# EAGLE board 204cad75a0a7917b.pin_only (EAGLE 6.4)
REV: B

Size 50.8 x 22.86 mm. Coordinates in mm from the lower left corner, seen from the top.
Outline: 2.54,0 48.26,0 arc90 50.8,2.54 50.8,20.32 arc90 48.26,22.86 2.54,22.86 arc90 0,20.32 0,13.97 0.51,13.46 0.51,9.4 0,8.89 0,2.54 arc90 2.54,0
Copper layers (1*16): Top 0.035mm / dielectric 1.5mm / Bottom 0.035mm
Design rules "adafruit *": minimum track width 8mil, minimum drill 15.5mil, track to track 8mil, track to pad 8mil, pad to pad 8mil, via to via 8mil, smd to smd 8mil, copper to edge 10mil, drill to drill 8mil, minimum pad ring 10mil, minimum via ring 8mil, stop-mask expansion 2mil, vias tented up to drill 20mil, thermal gap 10mil
Holes 2.54 mm at 48.26,20.32 48.26,2.54
tRestrict: area 20.8,9.3 to 21.1,12.8; area 20.7,8.1 to 22.9,8.5; area 26.2,10.3 to 26.5,13.3

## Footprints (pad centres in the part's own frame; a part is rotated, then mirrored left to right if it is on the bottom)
1X01_ROUND = drill 1 pad 1.676: 1 0,0
0805-NO = smd 1.24 x 1.5: 1 -0.95,0; 2 0.95,0
0603-NO = smd 1.1 x 1: 1 -0.85,0; 2 0.85,0
_0603MP = smd 0.8 x 0.8: 1 -0.762,0; 2 0.762,0
CHIPLED_0805_NOOUTLINE = smd 1.2 x 1.2: A 0,-1.05; C 0,1.05
SOD-123 = smd 1.4 x 1.4: A 1.85,0; C -1.85,0
TQFN44_7MM = smd 0.25 x 0.8: 1 -2.5,-3.475; 2 -2,-3.475; 3 -1.5,-3.475; 4 -1,-3.475; 5 -0.5,-3.475; 6 0,-3.475; 7 0.5,-3.475; 8 1,-3.475; 9 1.5,-3.475; 10 2,-3.475; 11 2.5,-3.475; 23 2.5,3.475; 24 2,3.475; 25 1.5,3.475; 26 1,3.475; 27 0.5,3.475; 28 0,3.475; 29 -0.5,3.475; 30 -1,3.475; 31 -1.5,3.475; 32 -2,3.475; 33 -2.5,3.475 | smd 0.8 x 0.25: 12 3.475,-2.5; 13 3.475,-2; 14 3.475,-1.5; 15 3.475,-1; 16 3.475,-0.5; 17 3.475,0; 18 3.475,0.5; 19 3.475,1; 20 3.475,1.5; 21 3.475,2; 22 3.475,2.5; 34 -3.475,2.5; 35 -3.475,2; 36 -3.475,1.5; 37 -3.475,1; 38 -3.475,0.5; 39 -3.475,0; 40 -3.475,-0.5; 41 -3.475,-1; 42 -3.475,-1.5; 43 -3.475,-2; 44 -3.475,-2.5 | smd 4.7 x 4.7: THERMAL 0,0
1X16_ROUND = drill 1 pad 1.676: 1 -19.05,0; 2 -16.51,0; 3 -13.97,0; 4 -11.43,0; 5 -8.89,0; 6 -6.35,0; 7 -3.81,0; 8 -1.27,0; 9 1.27,0; 10 3.81,0; 11 6.35,0; 12 8.89,0; 13 11.43,0; 14 13.97,0; 15 16.51,0; 16 19.05,0
1X12_ROUND = drill 1 pad 1.676: 1 -13.97,0; 2 -11.43,0; 3 -8.89,0; 4 -6.35,0; 5 -3.81,0; 6 -1.27,0; 7 1.27,0; 8 3.81,0; 9 6.35,0; 10 8.89,0; 11 11.43,0; 12 13.97,0
1X02_ROUND = drill 1 pad 1.778: 1 -1.27,0; 2 1.27,0
KMR2 = smd 1 x 1: 1 2,0.8; 2 2,-0.8; 3 -2,0.8; 4 -2,-0.8
SOT23-5 = smd 0.55 x 1.2: 1 -0.95,-1.3; 2 0,-1.3; 3 0.95,-1.3; 4 0.95,1.3; 5 -0.95,1.3
RFMHCW_SMT = smd 1.5 x 1: 1P 8.1,-7; 2P 8.1,-5; 3P 8.1,-3; 4P 8.1,-1; 5P 8.1,1; 6P 8.1,3; 7P 8.1,5; 8P 8.1,7; 9P -8.1,7; 10P -8.1,5; 11P -8.1,3; 12P -8.1,1; 13P -8.1,-1; 14P -8.1,-3; 15P -8.1,-5; 16P -8.1,-7
MOUNTINGHOLE_2.5_PLATED = drill 2.5 pad 3.2: P$1 0,0
FIDUCIAL_1MM = smd 1 x 1: 1 0,0
JSTPH2 = smd 1 x 4.6: 1 -1,-3.7; 2 1,-3.7 | smd 1.6 x 3.4: NC1 -3.4,1.5; NC2 3.4,1.5
U.FL = smd 2.2 x 1.05: 1 0,1.375; 2 0,-1.375 | smd 0.8 x 1: 3 1.525,0
4UCONN_20329_V2 = smd 1 x 2: BASE@1 -0.75,-2; BASE@2 0.75,-2 | smd 0.4 x 1.35: D+ 0,0.775; D- -0.65,0.775; GND 1.3,0.775; ID 0.65,0.775; VBUS -1.3,0.775 | drill 0.8 pad 1.2 offset: SPRT@1 -3.3,0.9; SPRT@2 3.3,0.9 | drill 0.9 pad 2.5 square: SPRT@3 -3.6,-1.9; SPRT@4 3.6,-1.9 | hole 0.7: -1.95,0; 1.95,0
RESONATOR-SMD = smd 0.7 x 1.7: 1 -1.2,0; 2 0,0; 3 1.2,0

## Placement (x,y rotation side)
ANT  [1X01_ROUND]  49.53,5.46 0 top
C1  10uF  [0805-NO]  49.59,9.4 270 top
C3  10µF  [0805-NO]  11.81,12.06 0 top
C6  10µF  [0805-NO]  8.09,12.96 90 top
C7  1uF  [0603-NO]  19.07,15.29 90 top
C8  10µF  [0805-NO]  14.37,11.62 270 top
C9  1uF  [_0603MP]  27.29,15.48 315 top
C14  1uF  [0603-NO]  10.59,4.09 0 top
CHG  ORANGE  [CHIPLED_0805_NOOUTLINE]  2.41,5.59 270 top
D4  MBR120  [SOD-123]  17.91,18.92 180 top
IC1  ATMEGA32U4-MU  [TQFN44_7MM]  23.56,11.05 0 top
JP1  [1X16_ROUND]  25.4,1.27 180 top
JP3  [1X12_ROUND]  30.48,21.59 0 top
JP4  [1X02_ROUND]  49.53,13.97 90 top
L  RED  [CHIPLED_0805_NOOUTLINE]  2.65,17.36 90 top
R1  100k  [0603-NO]  49.97,17.91 270 top
R2  1K  [0603-NO]  6.22,4.19 0 top
R3  100k  [0603-NO]  28.32,17.91 180 top
R4  22  [0603-NO]  8.22,10.27 0 top
R5  22  [0603-NO]  8.15,8.88 0 top
R6  100K  [0603-NO]  29.21,15.56 270 top
R7  2.2K  [0603-NO]  5.59,20.95 270 top
R8  10K\  [0603-NO]  13.72,4.19 180 top
R9  100k  [0603-NO]  17.4,17.42 180 top
SW1  SPST_TACT-KMR2  [KMR2]  9.4,6.48 180 top
U2  AP2112-3.3  [SOT23-5]  16.56,14.81 180 top
U3  MCP73831T-2ACI/OT  [SOT23-5]  13.97,7.75 180 top
U4  [RFMHCW_SMT]  39.12,11.43 0 top
U$4  [ADAFRUIT_5MM]  2.67,13.84 180 bottom
U$5  [FEATHERLOGO]  30.61,4.83 0 bottom
U$6  [PCBFEAT-REV-040]  10.67,16.89 0 bottom
U$7  [ADAFRUIT_3.5MM]  20.32,19.18 270 top
U$31  MOUNTINGHOLE2.5  [MOUNTINGHOLE_2.5_PLATED]  2.54,20.32 270 top
U$32  MOUNTINGHOLE2.5  [MOUNTINGHOLE_2.5_PLATED]  2.54,2.54 270 top
U$34  FIDUCIAL""  [FIDUCIAL_1MM]  10.79,20.07 270 top
U$35  FIDUCIAL""  [FIDUCIAL_1MM]  46.4,1.02 270 top
X1  JSTPH  [JSTPH2]  10.67,19.3 0 top
X2  uFL  [U.FL]  47.18,6.22 180 bottom
X3  microUSB  [4UCONN_20329_V2]  4.45,11.43 270 top
Y1  8MHz  [RESONATOR-SMD]  28.06,5.39 180 top

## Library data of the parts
ANT C1 C3 C6 C7 C9 C14 CHG D4 IC1 JP1 JP3 JP4 L R1-R9 U2-U4 U$4-U$7 X1-X3 = microbuilder
C8 = microbuilder; COMPANY: ADAFRUIT INDUSTRIES; DRAWN: KTOWN; REV: A
SW1 = adafruit
U$31 U$32 U$34 U$35 = microbuilder; BOM: EXCLUDE
Y1 = SparkFun

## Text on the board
tPlace: 3 | 2 | BAT | En | USB | 13 | 12 | ~11 | ~ | 10 | ~ | 9 | ~ | 6 | ~ | 5 | SCL | SDA | #13 | 2 | 3 | RST | adafruit | Feather | 32u4 | RFM69HCW | RFMHCW | CHG | RST | 3V | ARf | GND | A0 | A1 | A2 | A3 | A4 | A5 | SCK | MO | MI | RX | TX | IO1 | 0 | 1
bPlace: 3 | 2 | 3.7/4.2V / LiPoly Batt / µUSB charge | En | 13 | 12 | ~ | 11 | ~ | 10 | ~ | 9 | 6 | ~ | 5 | SCL | SDA | BAT | USB | Feather 32u4 / RFM69HCW Radio | Node# | ATmega32u4 / 8MHz & 3.3V | RF Radio uses: / MISO/MOSI/SCK (SPI) / 4(RST), 7(IRQ), 8(CS) | Ant. | Freq | +20dBm | SCK | MOSI | MISO | RST | 3V | Aref | GND | A0 | A1 | A2 | A3 | A4 | A5 | RX | TX | IO1 | 0 | 1

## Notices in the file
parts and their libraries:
microbuilder: This work is placed in the public domain, and may be freely used for commercial and non-commercial work with the following conditions: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
SparkFun: Licensing: CC v3.0 Share-Alike You are welcome to use this library for commercial purposes.
